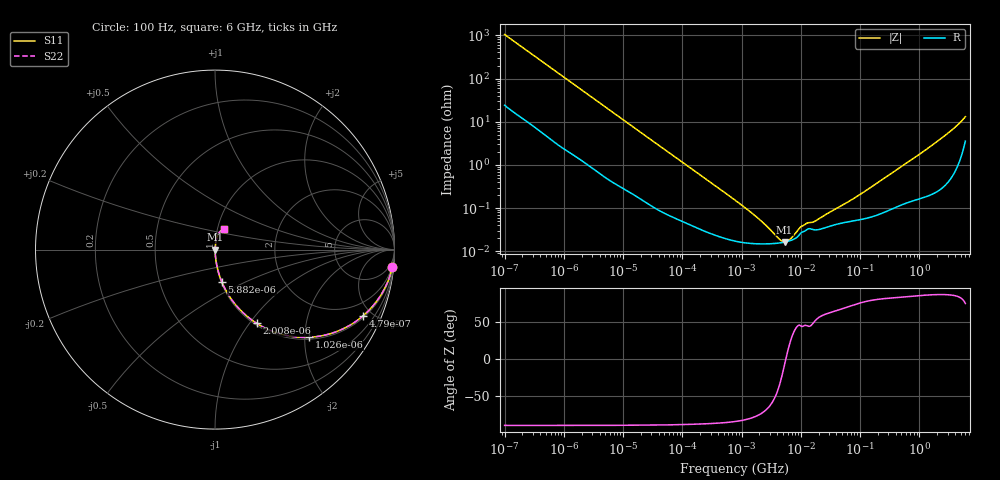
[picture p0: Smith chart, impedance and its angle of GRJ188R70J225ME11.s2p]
!Murata Part Number: GRJ188R70J225ME11
!These Parameters are Measured in Series Mode Connection
!Data Generated on Jun 19, 2026
!  o--ll--o
!Port1  Port2
!  o------o
!Operation Temp=25[degC], DC Bias Voltage=0[V]
!Freq. Start=100[Hz] Stop=6[GHz] 401[Steps]
# Hz S RI R 50
!Freq.(Hz) S11(Real) S11(Imag) S21(Real) S21(Imag) S12(Real) S12(Imag) S22(Real) S22(Imag)
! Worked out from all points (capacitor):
!   401 points, 100 Hz to 6 GHz, reference 50 ohm
!   read as one part in series: C = 1.52 uF near 109 Hz
!   lowest |Z| = 16.6 mohm at 5.312 MHz (marker M1)
!   series resonance near 5.592 MHz, so ESL is about 530 pH
!   S11 on the Smith chart (normalised r, x): 100 Hz: 1, -21; 479 Hz: 1.10, -4.45; 1.026 kHz: 1.05, -2.10; 2.008 kHz: 1.03, -1.08; 5.882 kHz: 1.01, -0.38; 6 GHz: 1.07, +0.25
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100  0.9888 -0.0944  0.0112 0.0944  0.0112 0.0944  0.9888 -0.0944
245  0.9446 -0.2176  0.0554 0.2176  0.0554 0.2176  0.9446 -0.2176
479  0.8269 -0.3675  0.1731 0.3675  0.1731 0.3675  0.8269 -0.3675
686  0.7058 -0.445  0.2942 0.445  0.2942 0.445  0.7058 -0.445
1026  0.5241 -0.4886  0.4759 0.4886  0.4759 0.4886  0.5241 -0.4886
1404  0.3756 -0.4731  0.6244 0.4731  0.6244 0.4731  0.3756 -0.4731
2008  0.2322 -0.4108  0.7678 0.4108  0.7678 0.4108  0.2322 -0.4108
3287  0.1057 -0.296  0.8943 0.296  0.8943 0.296  0.1057 -0.296
5882  0.038 -0.1799  0.962 0.1799  0.962 0.1799  0.038 -0.1799
13772  0.00872 -0.0803  0.9913 0.0803  0.9913 0.0803  0.00872 -0.0803
40335  0.00168 -0.0282  0.9983 0.0282  0.9983 0.0282  0.00168 -0.0282
774597  0.000176 -0.00153  0.9998 0.00153  0.9998 0.00153  0.000176 -0.00153
1983483  0.00015 -0.000537  0.9999 0.000537  0.9999 0.000537  0.00015 -0.000537
4440638  0.000158 -0.000102  0.9998 0.000102  0.9998 0.000102  0.000158 -0.000102
5311619  0.000164 -2.25e-05  0.9998 2.25e-05  0.9998 2.25e-05  0.000164 -2.25e-05
6644369  0.000178 7.62e-05  0.9998 -7.62e-05  0.9998 -7.62e-05  0.000178 7.62e-05
1.039699e7  0.00028 0.000264  0.9997 -0.000264  0.9997 -0.000264  0.00028 0.000264
1.555665e7  0.000325 0.000341  0.9997 -0.000341  0.9997 -0.000341  0.000325 0.000341
7.455971e7  0.000507 0.00153  0.9995 -0.00153  0.9995 -0.00153  0.000507 0.00153
3.124326e8  0.000937 0.00586  0.9991 -0.00586  0.9991 -0.00586  0.000937 0.00586
1.95892e9  0.00353 0.0339  0.9965 -0.0339  0.9965 -0.0339  0.00353 0.0339
6e9  0.0485 0.1156  0.9515 -0.1156  0.9515 -0.1156  0.0485 0.1156
